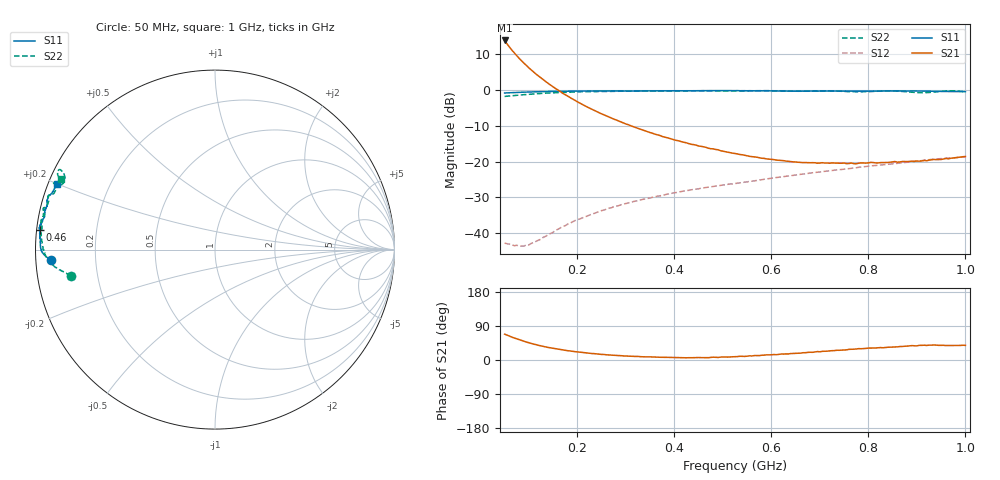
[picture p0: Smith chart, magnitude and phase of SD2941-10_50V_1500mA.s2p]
!Agilent Technologies,E8358A,US42080673,A.04.86
!Agilent E8358A: A.04.86
!Date: Friday, June 09, 2006 14:41:59
!Correction: S11(Full 2 Port SOLT,1,2) S21(Full 2 Port SOLT,1,2) S12(Full 2 Port SOLT,1,2) S22(Full 2 Port SOLT,1,2)
!S2P File: Measurements: S11, S21, S12, S22:
# Hz S  MA  R 50
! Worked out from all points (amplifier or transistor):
!   191 points, 50 MHz to 1 GHz, reference 50 ohm
!   highest |S21| = 13.9 dB at 50 MHz (marker M1)
!   |S21| within 3 dB of that: start of sweep to 66.8 MHz
!   unconditionally stable (mu >= 1): 770.6 MHz to 798.2 MHz; 880.7 MHz to 955.2 MHz; 991.6 MHz to end of sweep
!   at 205 MHz: K = 0.41, MSG = 16.2 dB, |S12| = -36.1 dB
!   at 525 MHz: K = 0.35, MSG = 4.2 dB, |S12| = -26.2 dB
!   at 1 GHz: K = 1.07, MAG = -1.6 dB, |S12| = -18.6 dB
!   S11 on the Smith chart (normalised r, x): 50 MHz: 0.05, -0.03; 460 MHz: 0.01, +0.06; 1 GHz: 0.02, +0.20
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5e7  0.9129 -176.4  4.971 68.2  0.007177 13.5  0.816 -169.7
5.5e7  0.9156 -176.5  4.445 65.8  0.007047 15.0  0.8235 -170.1
6e7  0.9201 -176.7  4.017 62.9  0.006907 17.5  0.8273 -170.4
6.5e7  0.9204 -176.9  3.634 60.3  0.006816 21.4  0.8347 -170.7
7.5e7  0.9274 -177.1  3.034 55.6  0.006701 26.7  0.8466 -171.2
8.5e7  0.9347 -177.3  2.581 51.2  0.006515 34.9  0.8572 -171.9
1e8  0.9415 -177.7  2.053 45.5  0.006777 44.9  0.8745 -172.6
1.1e8  0.947 -177.9  1.795 41.9  0.007325 51.4  0.8848 -173.1
1.2e8  0.95 -178.2  1.577 38.7  0.007913 57.6  0.8937 -173.6
1.4e8  0.958 -178.9  1.241 33.1  0.009455 66.9  0.9113 -174.8
1.7e8  0.965 -179.6  0.903 26.7  0.01231 74.2  0.9318 -176.5
2.1e8  0.9725 179.4  0.6319 19.8  0.0162 77.5  0.9525 -178.6
2.75e8  0.9743 177.5  0.3932 12.5  0.02322 79.3  0.9625 178.2
3.7e8  0.9792 175.7  0.2317 7.2  0.03295 78.1  0.9733 174.2
4.6e8  0.9822 173.5  0.1609 6.3  0.0427 75.6  0.9824 170.6
5.25e8  0.9832 172.3  0.1295 8.8  0.04913 74.1  0.9711 168.6
6.85e8  0.9722 168.1  0.09632 20.3  0.0696 69.8  0.9719 162.9
7.9e8  0.9671 165.3  0.09519 30.1  0.08439 66.7  0.9485 159.1
8.45e8  0.974 163.7  0.09783 33.9  0.09195 65.1  0.9767 157.5
9e8  0.9736 162.1  0.1017 37.3  0.1011 63.4  0.925 156.8
9.6e8  0.9583 159.7  0.1105 38.2  0.1111 61.0  0.9757 152.8
1e9  0.9544 157.5  0.1175 38.6  0.1168 57.5  0.9454 155.6
